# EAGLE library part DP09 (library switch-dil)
DIL/CODE SWITCH
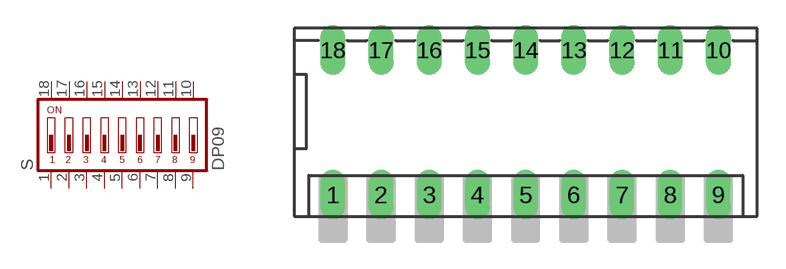
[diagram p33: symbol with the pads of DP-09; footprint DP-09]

Designator prefix S

## DP09 (MPN: MCDP09; OC_FARNELL: 1522007; OC_NEWARK: 74M2979)  [DP-09]
1  1  pas
2  2  pas
3  3  pas
4  4  pas
5  5  pas
6  6  pas
7  7  pas
8  8  pas
9  9  pas
10  10  pas
11  11  pas
12  12  pas
13  13  pas
14  14  pas
15  15  pas
16  16  pas
17  17  pas
18  18  pas

## Footprint DP-09 (pad centres in mm)
DIL/CODE SWITCH
drill 0.813 long: 1 -10.16,-3.81; 2 -7.62,-3.81; 3 -5.08,-3.81; 4 -2.54,-3.81; 5 0,-3.81; 6 2.54,-3.81; 7 5.08,-3.81; 8 7.62,-3.81; 9 10.16,-3.81; 10 10.16,3.81; 11 7.62,3.81; 12 5.08,3.81; 13 2.54,3.81; 14 0,3.81; 15 -2.54,3.81; 16 -5.08,3.81; 17 -7.62,3.81; 18 -10.16,3.81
